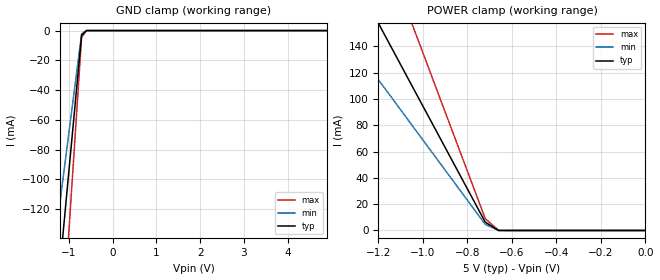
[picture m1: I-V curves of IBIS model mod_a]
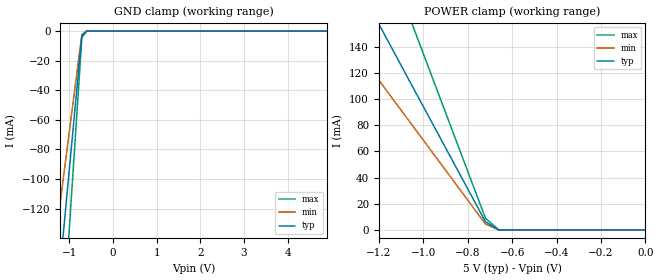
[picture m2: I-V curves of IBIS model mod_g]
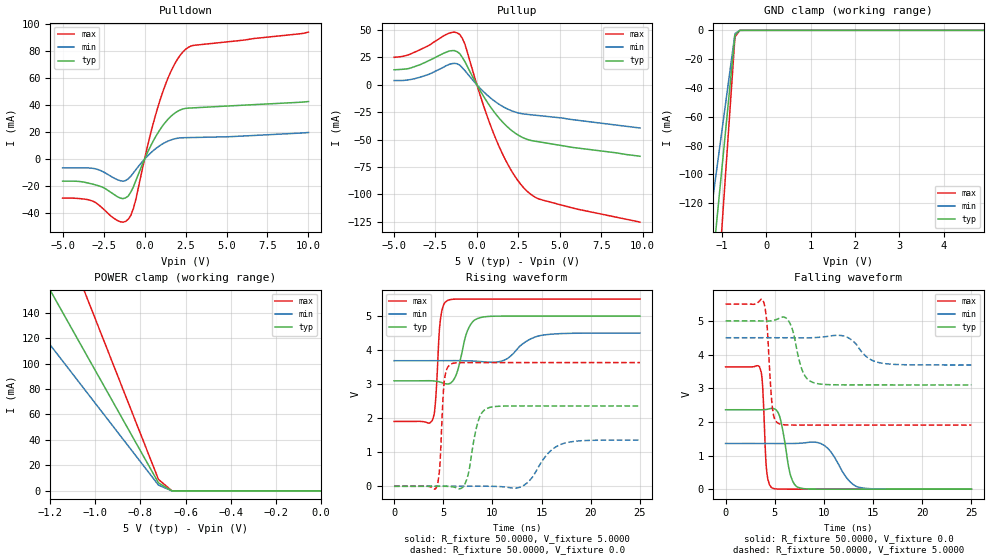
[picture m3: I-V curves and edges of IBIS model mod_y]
| IBIS (I/O, Buffer, Information, Specification) Model, officially
| electronic behavioral standard for Buffer structures of digital pins.
[IBIS ver]  4.0
[File name] 54hc138_5v0_rev1.ibs
[File Rev]  1.0
[Date]   27 Feb 2019
[Source]   CAD & Design Services (Catania) - STMicroelectronics
[Notes]
  (Note1) This IBIS model is the model of the product with package
   (Flat16 package elements);
  (Note2) This IBIS model is extracted with nominal 5.0V power supply
   (min:4.5V, typ:5.0V, max:5.5V);
  (Note3) This model has few Warnings about the non-monotonicity
   of I-V curves, but they are not indicative of problems
   inside the model;
[Disclaimer]
   Customers are solely responsible for all aspects of their
   own product designs or applications using this IBIS Model.
   STMicroelectronics assumes no liability for Custmer Designs
   and applications associated to this IBIS Model.
   In the use of this IBIS Model Customer shall not modify,
   disassemble, alter this Model in whole or in part.
   If Customers do not accept these terms, the IBIS Model
   may not be used. For any problems or modifications please
   contact STMicroelectronics (www.st.com).
[Copyright] (c) 2019 STMicroelectronics
|   Component 54HC138
[Component] 54HC138
[Manufacturer] STMicroelectronics
[Package]
| variable  typ   min   max
R_pkg   0.0   0.0   0.0
L_pkg   0.0H   0.0H   0.0H
C_pkg   0.0F   0.0F   0.0F
[Pin]  signal_name   model_name   R_pin   L_pin   C_pin
1   A   mod_a   87.8m   2.68nH   1.16pF
2   B   mod_a   53.6m   1.94nH   1.11pF
3   C   mod_a   34.1m   1.02nH   0.87pF
4   G2AN   mod_g   34.1m   1.02nH   0.87pF
5   G2BN   mod_g   34.1m   1.02nH   0.87pF
6   G1   mod_g   34.1m   1.02nH   0.87pF
7   Y7N   mod_y   53.6m   1.94nH   1.11pF
8   VSS   GND   87.8m   2.68nH   1.16pF
9   Y6N   mod_y   87.8m   2.68nH   1.16pF
10   Y5N   mod_y   53.6m   1.94nH   1.11pF
11   Y4N   mod_y   34.1m   1.02nH   0.87pF
12   Y3N   mod_y   34.1m   1.02nH   0.87pF
13   Y2N   mod_y   34.1m   1.02nH   0.87pF
14   Y1N   mod_y   34.1m   1.02nH   0.87pF
15   Y0N   mod_y   53.6m   1.94nH   1.11pF
16   VDD   POWER   87.8m   2.68nH   1.16pF
| Models and submodels in the file (3): mod_a (Input), mod_g (Input), mod_y (I/O)
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|   Model mod_a
[Model]   mod_a
Model_type  Input
Vinl   =   1.500V
Vinh   =   3.500V
C_comp   1.112pF   1.062pF   1.164pF
[Temperature Range]  25.0000   0.1250k   -55.0000
[Voltage Range]   5.0000V   4.5000V   5.5000V
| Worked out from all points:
|   GND clamp passes 1 mA (typ) near -0.63 V on its own axis
|   POWER clamp passes 1 mA (typ) near -0.67 V on its own axis
[GND_clamp]
|Voltage   I(typ)   I(min)   I(max)
-5V       -1.352A    -988.3mA   -1.933A
-1.37V    -210.9mA   -153.4mA   -301.2mA
-1.26V    -176.3mA   -128.3mA   -251.8mA
-1.15V    -141.7mA   -103.1mA   -202.3mA
-1.04V    -107mA     -77.87mA   -152.9mA
-930mV    -72.41mA   -52.68mA   -103.4mA
-710mV    -3.148mA   -2.29mA    -4.496mA
-600mV    -4.415uA   -5.303uA   -26.1uA
4.9V      7.144nA    7.624nA    8.792nA
[POWER_clamp]
|Voltage   I(typ)   I(min)   I(max)
-4.98V    1.347A     980.3mA    1.924A
-1.38V    214.1mA    155.7mA    305.7mA
-1.32V    195.2mA    142mA      278.7mA
-1.2V     157.4mA    114.5mA    224.8mA
-1.14V    138.5mA    100.8mA    197.8mA
-1.08V    119.6mA    87.03mA    170.8mA
-1.02V    100.7mA    73.29mA    143.9mA
-720mV    6.297mA    4.581mA    8.992mA
-660mV    1.654uA    640.4nA    66.12uA
0V        0A         0A         0A
|   Model mod_g
[Model]   mod_g
Model_type  Input
Vinl   =   1.500V
Vinh   =   3.500V
C_comp   0.925pF   0.883pF   0.968pF
[Temperature Range]  25.0000   0.1250k   -55.0000
[Voltage Range]   5.0000V   4.5000V   5.5000V
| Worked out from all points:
|   GND clamp passes 1 mA (typ) near -0.63 V on its own axis
|   POWER clamp passes 1 mA (typ) near -0.67 V on its own axis
[GND_clamp]
|Voltage   I(typ)   I(min)   I(max)
-5V       -1.352A    -988.3mA   -1.933A
-1.37V    -210.9mA   -153.4mA   -301.2mA
-1.26V    -176.3mA   -128.3mA   -251.8mA
-1.15V    -141.7mA   -103.1mA   -202.3mA
-1.04V    -107mA     -77.87mA   -152.9mA
-930mV    -72.41mA   -52.68mA   -103.4mA
-710mV    -3.148mA   -2.29mA    -4.496mA
-600mV    -4.415uA   -5.303uA   -26.1uA
4.9V      7.144nA    7.624nA    8.792nA
[POWER_clamp]
|Voltage   I(typ)   I(min)   I(max)
-4.98V    1.347A     980.3mA    1.924A
-1.38V    214.1mA    155.7mA    305.7mA
-1.32V    195.2mA    142mA      278.7mA
-1.2V     157.4mA    114.5mA    224.8mA
-1.14V    138.5mA    100.8mA    197.8mA
-1.08V    119.6mA    87.03mA    170.8mA
-1.02V    100.7mA    73.29mA    143.9mA
-720mV    6.297mA    4.581mA    8.992mA
-660mV    1.654uA    640.4nA    66.12uA
0V        0A         0A         0A
|   Model mod_y
[Model]   mod_y
Model_type I/O
Polarity   Non-Inverting
Vinl   =   1.500V
Vinh   =   3.500V
Vmeas  =   2.500V
Cref   =   50pF
C_comp   2.433pF   2.323pF   2.668pF
[Temperature Range]  25.0000   0.1250k   -55.0000
[Voltage Range]   5.0000V   4.5000V   5.5000V
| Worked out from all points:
|   slope of the pulldown table from 0 to 0.75 V, typ, clamps not added: 41.3 ohm
|   slope of the pullup table from 0 to 0.75 V, typ, clamps not added: 40.1 ohm
|   GND clamp passes 1 mA (typ) near -0.63 V on its own axis
|   POWER clamp passes 1 mA (typ) near -0.67 V on its own axis
|   rising waveform, R_fixture 50.0000, V_fixture 5.0000: 20-80 % time 999ps typ, 2.01ns min, 421ps max; typ from 3.1 V to 5 V
|   rising waveform, R_fixture 50.0000, V_fixture 0.0: 20-80 % time 900ps typ, 2.03ns min, 365ps max; typ from 0 V to 2.36 V
|   falling waveform, R_fixture 50.0000, V_fixture 0.0: 20-80 % time 826ps typ, 1.73ns min, 327ps max; typ from 2.36 V to 0 V
|   falling waveform, R_fixture 50.0000, V_fixture 5.0000: 20-80 % time 954ps typ, 1.57ns min, 452ps max; typ from 5 V to 3.1 V
[Pulldown]
|Voltage   I(typ)   I(min)   I(max)
-5V       -16.29mA   -6.393mA   -28.8mA
-3.24V    -18.23mA   -6.656mA   -30.69mA
-2.44V    -21.48mA   -9.875mA   -37.66mA
-1.64V    -27.88mA   -15.27mA   -45.52mA
-1.32V    -29.21mA   -16.31mA   -46.63mA
-1V       -27.39mA   -14.57mA   -44.52mA
-680mV    -20.51mA   -10.16mA   -36.49mA
280mV     7.467mA    3.521mA    14.58mA
1.08V     24.27mA    11.15mA    48.62mA
1.88V     34.37mA    15.18mA    71.36mA
2.68V     37.78mA    15.95mA    82.8mA
10V       42.63mA    19.74mA    94.02mA
[Pullup]
|Voltage   I(typ)   I(min)   I(max)
-5V       13.72mA    3.886mA    25.07mA
-3.44V    18.27mA    6.914mA    32mA
-1.68V    30.75mA    18.61mA    47.12mA
-1.04V    28.48mA    18.04mA    46.01mA
-720mV    21.01mA    12.89mA    36.98mA
400mV     -10.48mA   -6.279mA   -19.05mA
1.2V      -27.87mA   -16.35mA   -51.47mA
2V        -40.51mA   -23.12mA   -76.31mA
2.96V     -49.41mA   -26.87mA   -96.12mA
3.6V      -51.69mA   -27.88mA   -103.3mA
4.08V     -52.89mA   -28.64mA   -105.7mA
9.84V     -65.25mA   -39.43mA   -125.4mA
[GND_clamp]
|Voltage   I(typ)   I(min)   I(max)
-5V       -1.352A    -988.3mA   -1.933A
-1.37V    -210.9mA   -153.4mA   -301.2mA
-1.26V    -176.3mA   -128.3mA   -251.8mA
-1.15V    -141.7mA   -103.1mA   -202.3mA
-1.04V    -107mA     -77.87mA   -152.9mA
-930mV    -72.41mA   -52.68mA   -103.4mA
-710mV    -3.148mA   -2.29mA    -4.496mA
-600mV    -4.415uA   -5.303uA   -26.1uA
4.9V      7.144nA    7.624nA    8.792nA
[POWER_clamp]
|Voltage   I(typ)   I(min)   I(max)
-4.98V    1.347A     980.3mA    1.924A
-1.38V    214.1mA    155.7mA    305.7mA
-1.32V    195.2mA    142mA      278.7mA
-1.2V     157.4mA    114.5mA    224.8mA
-1.14V    138.5mA    100.8mA    197.8mA
-1.08V    119.6mA    87.03mA    170.8mA
-1.02V    100.7mA    73.29mA    143.9mA
-720mV    6.297mA    4.581mA    8.992mA
-660mV    1.654uA    640.4nA    66.12uA
0V        0A         0A         0A
[Ramp]
| variable   typ   min   max
dV/dt_r   1.4155/0.9977n   0.8146/2.1339n   2.1799/0.4424n
dV/dt_f   1.1414/1.0121n   0.4864/1.7261n   2.1568/0.5072n
R_load = 50.0000
[Rising Waveform]
R_fixture= 50.0000
V_fixture= 5.0000
V_fixture_min= 4.5000
V_fixture_max= 5.5000
|time   V(typ)   V(min)   V(max)
0s        3.098V     3.689V     1.905V
3.875ns   3.099V     3.689V     1.929V
4.225ns   3.089V     3.689V     2.532V
4.725ns   3.058V     3.69V      4.924V
5.425ns   3.004V     3.691V     5.456V
6.225ns   3.216V     3.691V     5.498V
7.425ns   4.54V      3.686V     5.5V
8.475ns   4.927V     3.672V     5.5V
15.15ns   5V         4.443V     5.5V
25ns      5V         4.5V       5.5V
[Rising Waveform]
R_fixture= 50.0000
V_fixture= 0.0
V_fixture_min= 0.0
V_fixture_max= 0.0
|time   V(typ)   V(min)   V(max)
0s        209.2pV    163.2pV    87.19pV
4.35ns    1.878mV    -51.02uV   -4.312mV
4.65ns    3.039mV    -75.04uV   589.3mV
5.1ns     2.372mV    -138.2uV   3.076V
5.95ns    -15.56mV   -6.381uV   3.611V
7.25ns    97.91mV    828.8uV    3.634V
9.45ns    2.288V     1.508mV    3.634V
13.2ns    2.36V      29.01mV    3.634V
17.4ns    2.36V      1.272V     3.634V
25ns      2.36V      1.357V     3.634V
[Falling Waveform]
R_fixture= 50.0000
V_fixture= 0.0
V_fixture_min= 0.0
V_fixture_max= 0.0
|time   V(typ)   V(min)   V(max)
0s        2.36V      1.358V     3.634V
3.45ns    2.359V     1.358V     3.636V
3.75ns    2.36V      1.357V     3.151V
4.2ns     2.371V     1.357V     490.7mV
4.725ns   2.401V     1.356V     38.66mV
5.5ns     2.163V     1.356V     2.121mV
7.4ns     52.62mV    1.362V     10.94uV
10.05ns   466.7uV    1.298V     10.47nV
13.5ns    4.665uV    59.25mV    -536.4pV
25ns      -59.62nV   16.98uV    -607.1pV
[Falling Waveform]
R_fixture= 50.0000
V_fixture= 5.0000
V_fixture_min= 4.5000
V_fixture_max= 5.5000
|time   V(typ)   V(min)   V(max)
0s        5V         4.5V       5.5V
3.875ns   4.997V     4.5V       5.562V
4.2ns     4.993V     4.5V       4.958V
4.775ns   5.01V      4.5V       2.386V
5.475ns   5.08V      4.5V       1.94V
6.55ns    4.927V     4.5V       1.907V
7.75ns    3.569V     4.497V     1.905V
8.9ns     3.17V      4.502V     1.905V
15.75ns   3.098V     3.751V     1.905V
25ns      3.098V     3.69V      1.905V
